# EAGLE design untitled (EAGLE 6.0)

## Sheet 1 of 3: NAP a SERVO
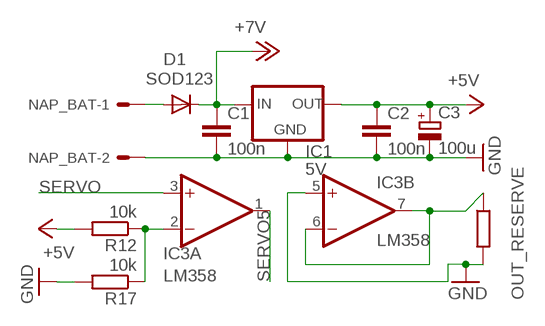
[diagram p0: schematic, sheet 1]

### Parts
C1  100n  C-EUC0805K  [C0805K]
C2  100n  C-EUC0805K  [C0805K]
C3  100u  CPOL-EUE2-5  [E2-5]
D1  SOD123  CGRM4001-G  [SOD-123_MINI-SMA]
IC1  5V  78XXL  [78XXL]
IC3  LM358  TL072D  [SO08]
NAP_BAT  22-27-2021-02  [6410-02]
OUT_RESERVE  R-EU_R0805  [R0805]
R12  10k  R-EU_R0805  [R0805]
R17  10k  R-EU_R0805  [R0805]

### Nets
+7V: C1.1 D1.C IC1.IN ; also sheet 2
GND: C1.2 C2.2 C3.- IC1.GND IC3.5(B:+IN) NAP_BAT.2 OUT_RESERVE.2 R17.2 ; also sheet 2,3
N$2: D1.A NAP_BAT.1
N$6: IC3.6(B:-IN) IC3.7(B:OUT) OUT_RESERVE.1
N$14: IC3.2(A:-IN) R12.1 R17.1
SERVO: IC3.3(A:+IN) ; also sheet 2
SERVO5: IC3.1(A:OUT) ; also sheet 2
VCC: C2.1 C3.+ IC1.OUT R12.2 ; supply symbol labelled +5V ; also sheet 2,3

## Sheet 2 of 3: HEADER_IO
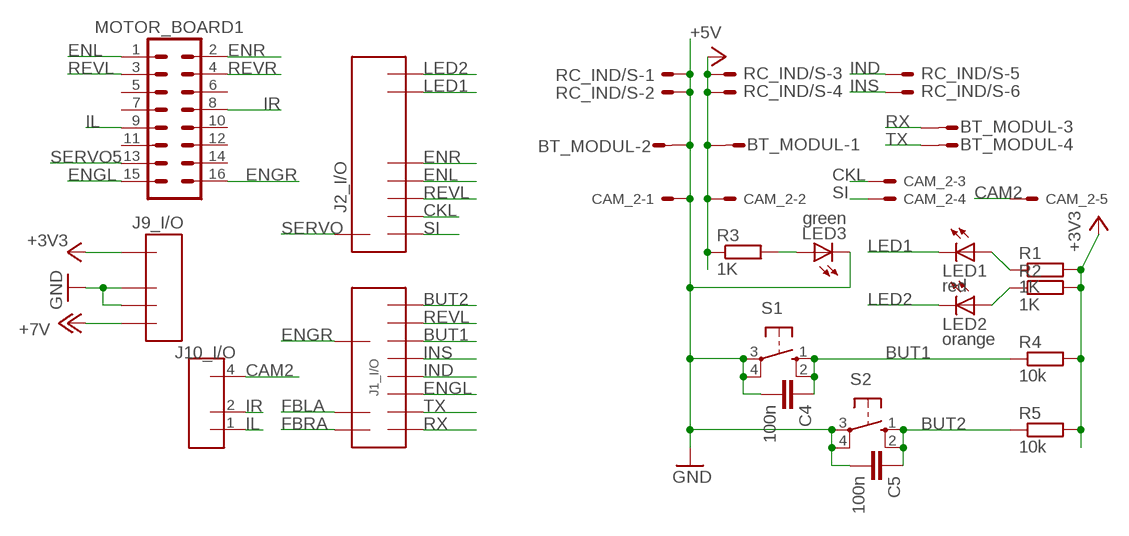
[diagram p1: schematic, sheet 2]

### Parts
BT_MODUL  M04S  [04P]
C4  100n  C-EUC0805K  [C0805K]
C5  100n  C-EUC0805K  [C0805K]
CAM_2  22-27-2051-05  [6410-05]
J1_I/O  DOLNE  [DOLNE]
J2_I/O  HORNE  [HORNE]
J9_I/O  NAP  [NAP]
J10_I/O  ANALOG  [ANALOG]
LED1  red  LED3MM  [LED3MM]
LED2  orange  LED3MM  [LED3MM]
LED3  green  LED3MM  [LED3MM]
MOTOR_BOARD1  ML16  [ML16]
R1  1K  R-EU_R0805  [R0805]
R2  1K  R-EU_R0805  [R0805]
R3  1K  R-EU_R0805  [R0805]
R4  10k  R-EU_R0805  [R0805]
R5  10k  R-EU_R0805  [R0805]
RC_IND/S  ML6E  [ML6]
S1  10-XX  [B3F-10XX]
S2  10-XX  [B3F-10XX]

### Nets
+3V3: J9_I/O.1 R1.2 R2.2 R4.2 R5.2
+7V: J9_I/O.4 ; also sheet 1
BUT1: C4.1 J1_I/O.P$9 R4.1 S1.1(S) S1.2(S1)
BUT2: C5.1 J1_I/O.P$11 R5.1 S2.1(S) S2.2(S1)
CAM2: CAM_2.5 J10_I/O.4
CKL: CAM_2.3 J2_I/O.P$3
ENGL: J1_I/O.P$5 MOTOR_BOARD1.15
ENGR: J1_I/O.P$8 MOTOR_BOARD1.16
ENL: J2_I/O.P$5 MOTOR_BOARD1.1
ENR: J2_I/O.P$6 MOTOR_BOARD1.2
FBLA: J1_I/O.P$3 ; also sheet 3
FBRA: J1_I/O.P$1 ; also sheet 3
GND: BT_MODUL.2 C4.2 C5.2 CAM_2.1 J9_I/O.2 J9_I/O.3 LED3.K(C) RC_IND/S.1 RC_IND/S.2 S1.3(P) S1.4(P1) S2.3(P) S2.4(P1) ; also sheet 1,3
IL: J10_I/O.1 MOTOR_BOARD1.9
IND: J1_I/O.P$6 RC_IND/S.5
INS: J1_I/O.P$7 RC_IND/S.6
IR: J10_I/O.2 MOTOR_BOARD1.8
LED1: J2_I/O.P$7 LED1.K(C)
LED2: J2_I/O.P$8 LED2.K(C)
N$1: LED1.A R1.1
N$15: LED2.A R2.1
N$16: LED3.A R3.2
REVL: J1_I/O.P$10 J2_I/O.P$4 MOTOR_BOARD1.3
REVR: MOTOR_BOARD1.4
RX: BT_MODUL.3 J1_I/O.P$2
SERVO: J2_I/O.P$1 ; also sheet 1
SERVO5: MOTOR_BOARD1.13 ; also sheet 1
SI: CAM_2.4 J2_I/O.P$2
TX: BT_MODUL.4 J1_I/O.P$4
VCC: BT_MODUL.1 CAM_2.2 R3.1 RC_IND/S.3 RC_IND/S.4 ; supply symbol labelled +5V ; also sheet 1,3
Unconnected: MOTOR_BOARD1.5 MOTOR_BOARD1.6 MOTOR_BOARD1.7 MOTOR_BOARD1.10 MOTOR_BOARD1.11 MOTOR_BOARD1.12 MOTOR_BOARD1.14

## Sheet 3 of 3: CNY70
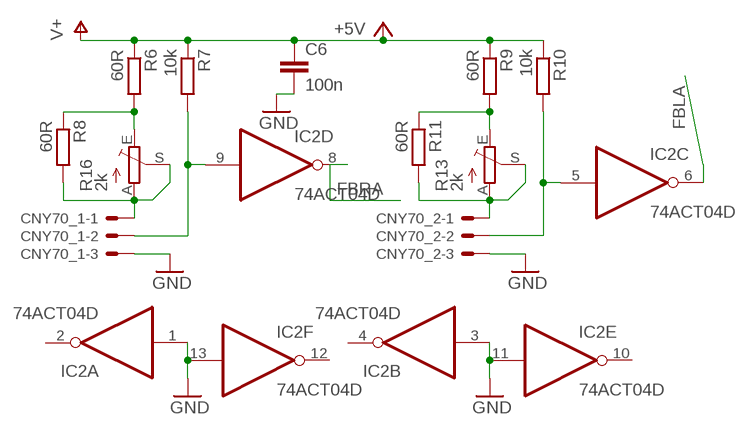
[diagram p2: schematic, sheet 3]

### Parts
C6  100n  C-EUC0805K  [C0805K]
CNY70_1  22-27-2031-03  [6410-03]
CNY70_2  22-27-2031-03  [6410-03]
IC2  74ACT04D  [SO14]
R6  60R  R-EU_R0603  [R0603]
R7  10k  R-EU_R0603  [R0603]
R8  60R  R-EU_R0603  [R0603]
R9  60R  R-EU_R0603  [R0603]
R10  10k  R-EU_R0603  [R0603]
R11  60R  R-EU_R0603  [R0603]
R13  2k  TRIM_EU-CA6V  [CA6V]
R16  2k  TRIM_EU-CA6V  [CA6V]

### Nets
FBLA: IC2.6(C:O) ; also sheet 2
FBRA: IC2.8(D:O) ; also sheet 2
GND: C6.2 CNY70_1.3 CNY70_2.3 IC2.1(A:I) IC2.3(B:I) IC2.11(E:I) IC2.13(F:I) ; also sheet 1,2
N$3: R9.2 R11.1 R13.E
N$4: R6.2 R8.1 R16.E
N$5: CNY70_2.1 R11.2 R13.A R13.S
N$8: CNY70_1.1 R8.2 R16.A R16.S
N$9: CNY70_1.2 IC2.9(D:I) R7.2
N$10: CNY70_2.2 IC2.5(C:I) R10.2
VCC: C6.1 R6.1 R7.1 R9.1 R10.1 ; supply symbol labelled V+, +5V ; also sheet 1,2
Unconnected: IC2.2(A:O) IC2.4(B:O) IC2.10(E:O) IC2.12(F:O)

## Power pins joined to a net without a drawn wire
GND: IC2.7(P:GND) IC3.4(P:V-)
VCC: IC2.14(P:VCC) IC3.8(P:V+)

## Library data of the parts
BT_MODUL = con-amp-quick:M04S: AMP QUICK CONNECTOR; OC_FARNELL: unknown; OC_NEWARK: unknown
C1 C2 C4-C6 = rcl:C-EU: CAPACITOR, European symbol
C3 = rcl:CPOL-EU: POLARIZED CAPACITOR, European symbol
CAM_2 = con-molex:22-?-05: CONNECTOR wire to board 2.54 mm (.1 inch) pitch header; OC_FARNELL: unknown; OC_NEWARK: unknown
CNY70_1 CNY70_2 = con-molex:22-?-03: CONNECTOR wire to board 2.54 mm (.1 inch) pitch header; OC_FARNELL: unknown; OC_NEWARK: unknown
D1 = diode:CGRM400*-G: Molded plasitc,JEDEC SOD-123/Mini SMA
IC1 = v-reg:78XXL: VOLTAGE REGULATOR
IC2 = 74xx-eu:74*04: Hex INVERTER
IC3 = linear:TL072: OP AMP
J1_I/O = con-tfc:DOLNE
J2_I/O = con-tfc:HORNE
J9_I/O = con-tfc:NAP
J10_I/O = con-tfc:ANALOG
LED1-LED3 = led:LED: LED
MOTOR_BOARD1 = con-ml:ML16: HARTING; OC_FARNELL: unknown; OC_NEWARK: unknown
NAP_BAT = con-molex:22-?-02: CONNECTOR; OC_FARNELL: unknown; OC_NEWARK: unknown
OUT_RESERVE R1-R12 R17 = rcl:R-EU_: RESISTOR, European symbol
R13 R16 = pot:TRIM_EU-: POTENTIOMETER
RC_IND/S = con-ml:ML6E: HARTING; OC_FARNELL: unknown; OC_NEWARK: unknown
S1 S2 = switch-omron:10-XX: OMRON SWITCH; MPN: B3F-1000; OC_FARNELL: 176432; OC_NEWARK: 36M3542

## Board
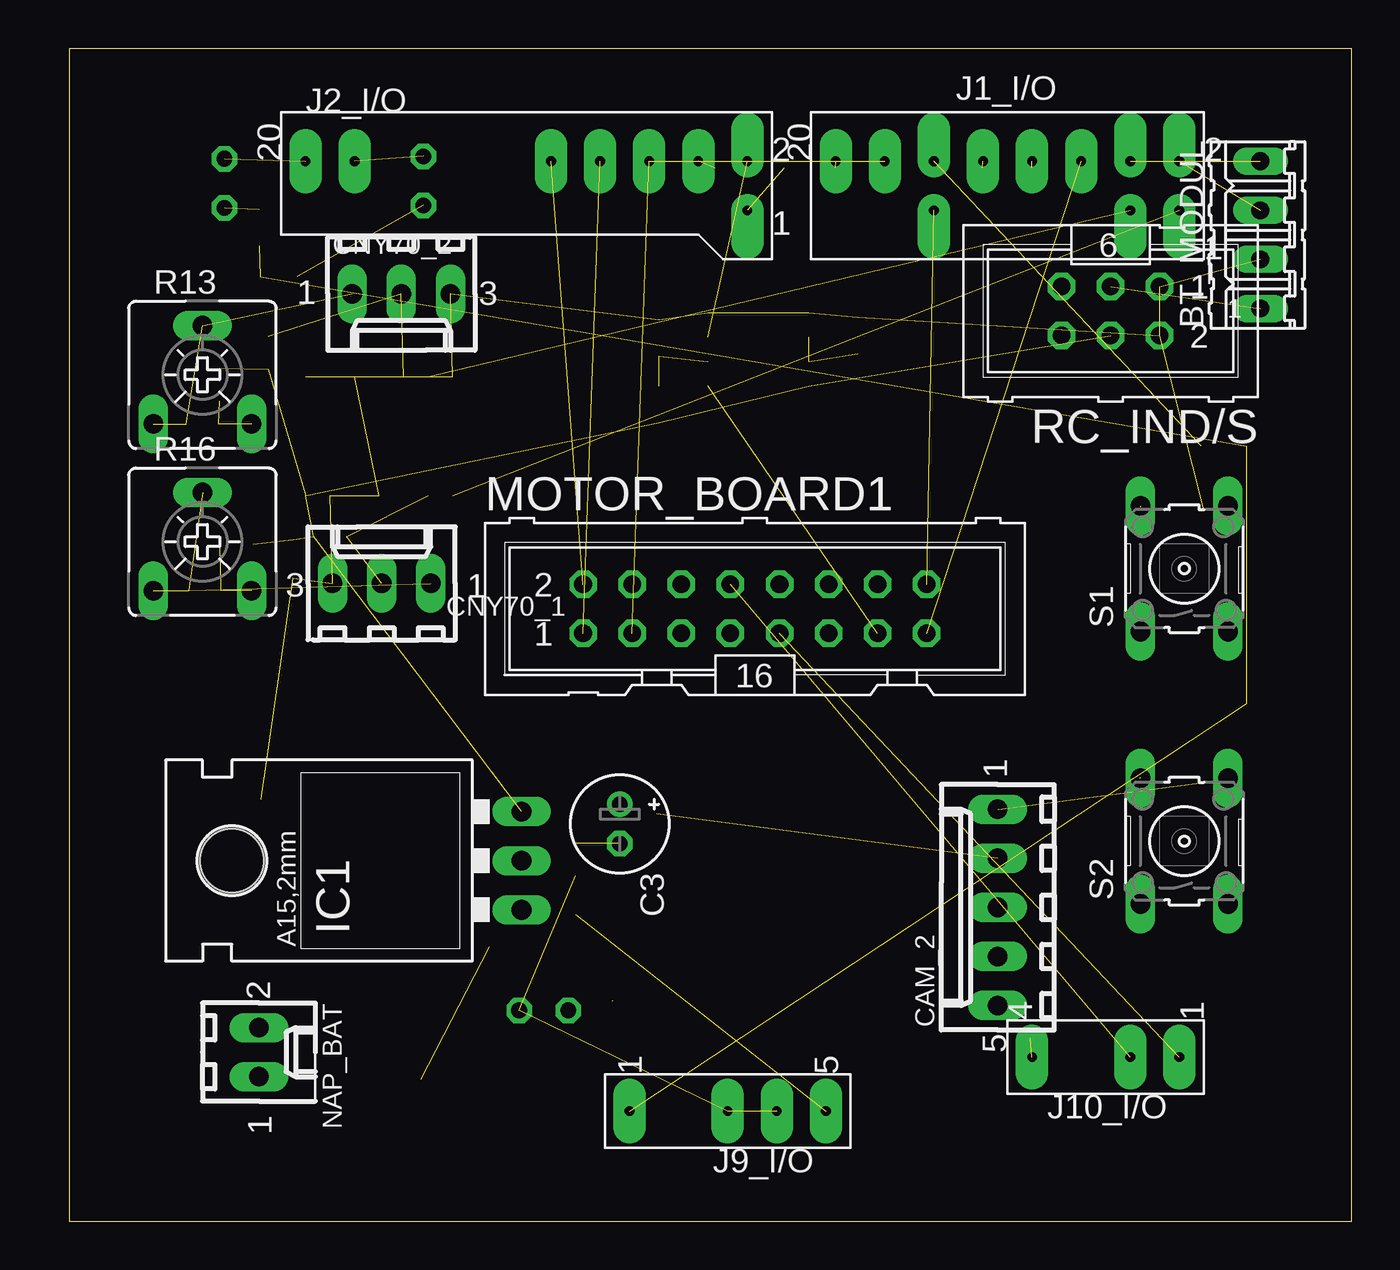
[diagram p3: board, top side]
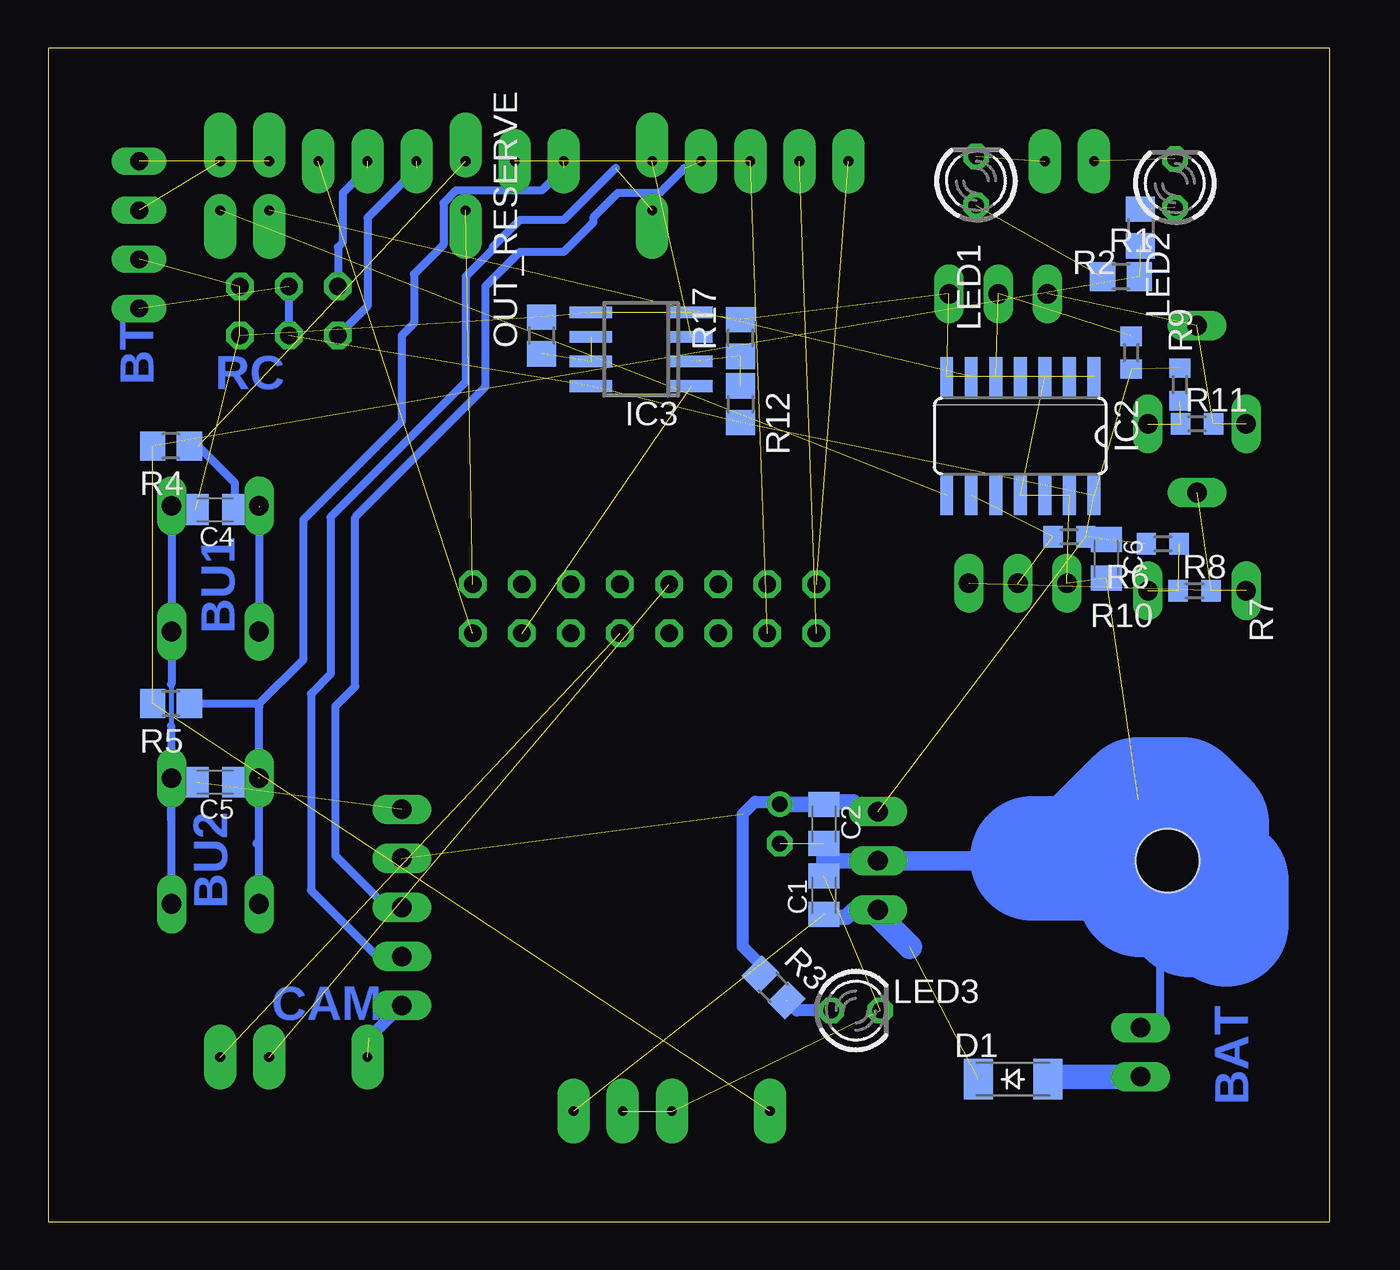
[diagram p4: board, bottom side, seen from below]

Size 66.29 x 60.71 mm. Coordinates in mm from the lower left corner, seen from the top.
Outline: 0,60.71 66.29,60.71 66.29,0 0,0 0,60.71
Copper layers (1*16): Top 0.035mm / dielectric 1.5mm / Bottom 0.035mm
Design rules: minimum track width 10mil, minimum drill 24mil, track to track 8mil, track to pad 8mil, pad to pad 8mil, via to via 8mil, smd to smd 8mil, copper to edge 40mil, drill to drill 8mil, minimum pad ring 10mil, minimum via ring 8mil, stop-mask expansion 4mil, vias tented up to drill 0mil, thermal gap 10mil

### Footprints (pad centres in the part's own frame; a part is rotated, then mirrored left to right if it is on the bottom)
04P = drill 0.914 long: 1 -3.81,0; 2 -1.27,0; 3 1.27,0; 4 3.81,0
C0805K = smd 1.3 x 1.6: 1 -1,0; 2 1,0
E2-5 = drill 0.813 pad 1.27: + -1.016,0 | drill 0.813 pad 1.27 octagon: - 1.016,0
6410-05 = drill 1.016 long: 1 5.08,0; 2 2.54,0; 3 0,0; 4 -2.54,0; 5 -5.08,0
6410-03 = drill 1.016 long: 1 2.54,0; 2 0,0; 3 -2.54,0
SOD-123_MINI-SMA = smd 1.5 x 2.1: A 1.8,0; C -1.8,0
78XXL = drill 1.016 long: GND 0,-3.81; IN -2.54,-3.81; OUT 2.54,-3.81 | hole 3.302: 0,11.176
SO14 = smd 0.66 x 2.032: 1 -3.81,-3.073; 2 -2.54,-3.073; 3 -1.27,-3.073; 4 0,-3.073; 5 1.27,-3.073; 6 2.54,-3.073; 7 3.81,-3.073; 8 3.81,3.073; 9 2.54,3.073; 10 1.27,3.073; 11 0,3.073; 12 -1.27,3.073; 13 -2.54,3.073; 14 -3.81,3.073
SO08 = smd 0.6 x 2.2: 1 -1.905,-2.6; 2 -0.635,-2.6; 3 0.635,-2.6; 4 1.905,-2.6; 5 1.905,2.6; 6 0.635,2.6; 7 -0.635,2.6; 8 -1.905,2.6
DOLNE = drill 0.5 pad 1.676 offset: P$1 8.89,-1.27; P$2 8.89,1.27; P$3 6.35,-1.27; P$4 6.35,1.27; P$8 -3.81,-1.27; P$9 -3.81,1.27 | drill 0.5 pad 1.676 long: P$5 3.81,1.27; P$6 1.27,1.27; P$7 -1.27,1.27; P$10 -6.35,1.27; P$11 -8.89,1.27
HORNE = drill 0.5 pad 1.676 offset: P$1 8.89,1.27; P$2 8.89,-1.27 | drill 0.5 pad 1.676 long: P$3 6.35,1.27; P$4 3.81,1.27; P$5 1.27,1.27; P$6 -1.27,1.27; P$7 -11.43,1.27; P$8 -13.97,1.27
NAP = drill 0.5 pad 1.676 long: 1 0,5.08; 2 0,0; 3 0,-2.54; 4 0,-5.08
ANALOG = drill 0.5 pad 1.676 long: 1 0,-3.81; 2 0,-1.27; 4 0,3.81
LED3MM = drill 0.813 octagon: A -1.27,0; K 1.27,0
ML16 = drill 0.914 octagon: 1 -8.89,-1.27; 2 -8.89,1.27; 3 -6.35,-1.27; 4 -6.35,1.27; 5 -3.81,-1.27; 6 -3.81,1.27; 7 -1.27,-1.27; 8 -1.27,1.27; 9 1.27,-1.27; 10 1.27,1.27; 11 3.81,-1.27; 12 3.81,1.27; 13 6.35,-1.27; 14 6.35,1.27; 15 8.89,-1.27; 16 8.89,1.27
6410-02 = drill 1.016 long: 1 1.27,0; 2 -1.27,0
R0805 = smd 1.3 x 1.5: 1 -0.95,0; 2 0.95,0
R0603 = smd 1 x 1.1: 1 -0.85,0; 2 0.85,0
CA6V = drill 1.016 long: A -2.54,-2.54; E 2.54,-2.54; S 0,2.54
ML6 = drill 0.914 octagon: 1 -2.54,-1.27; 2 -2.54,1.27; 3 0,-1.27; 4 0,1.27; 5 2.54,-1.27; 6 2.54,1.27
B3F-10XX = drill 1.016 long: 1 -3.251,2.261; 2 3.251,2.261; 3 -3.251,-2.261; 4 3.251,-2.261

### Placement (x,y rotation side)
BT_MODUL  61.6,51.05 90 top
C1  26.16,16.89 90 bottom
C2  26.16,20.57 270 bottom
C3  28.45,20.57 270 top
C4  57.66,36.83 180 bottom
C5  57.66,22.73 180 bottom
C6  11.56,34.29 270 bottom
CAM_2  48.01,16.26 90 top
CNY70_1  16.13,33.02 0 top
CNY70_2  17.14,48.01 180 top
D1  16.38,7.37 0 bottom
IC1  19.56,18.67 90 top
IC2  16,40.64 180 bottom
IC3  35.62,45.13 90 bottom
J1_I/O  48.51,53.59 0 top
J2_I/O  26.16,53.59 0 top
J9_I/O  34.04,5.71 90 top
J10_I/O  53.59,8.51 90 top
LED1  18.29,53.85 90 bottom
LED2  8,53.72 90 bottom
LED3  24.51,10.92 0 bottom
MOTOR_BOARD1  35.44,31.7 0 top
NAP_BAT  9.78,8.76 270 top
OUT_RESERVE  40.77,45.85 90 bottom
R1  10.79,48.89 0 bottom
R2  9.78,51.43 270 bottom
R3  28.78,12.12 315 bottom
R4  59.94,40.13 180 bottom
R5  59.94,26.8 180 bottom
R6  8.63,35.07 0 bottom
R7  13.46,35.43 180 bottom
R8  6.98,32.64 0 bottom
R9  7.75,43.31 270 bottom
R10  10.27,44.96 90 bottom
R11  6.86,41.27 0 bottom
R12  30.48,42.29 270 bottom
R13  6.86,43.81 0 top
R16  6.86,35.18 0 top
R17  30.48,45.72 90 bottom
RC_IND/S  53.85,47.12 180 top
S1  57.66,33.78 90 top
S2  57.66,19.69 90 top

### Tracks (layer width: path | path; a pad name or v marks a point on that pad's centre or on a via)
+3V3  (4 unrouted)
+7V  (2 unrouted)
  Bottom 0.813: IC1.IN 24.64,16.13 25.02,15.75 26.02,15.75 C1.1
  Bottom 1.27: IC1.IN 23.37,15.88 21.72,14.22
BUT1  (2 unrouted)
  Bottom 0.406: 55.37,36.96 55.5,36.83 C4.1 56.64,36.85 56.64,38.23 58.55,40.13 R4.1 | S1.2 S1.1
BUT2  (3 unrouted)
  Bottom 0.406: 39.6,54.5 40.77,53.34 45.21,53.34 45.85,52.7 45.85,50.55 47.37,49.02 47.37,46.48 48.01,45.85 48.01,41.4 53.09,36.32 53.09,29.08 55.37,26.8 55.37,26.67 | S2.1 55.4,19.69 | 55.4,19.69 S2.2 56.57,22.94 56.64,22.86 56.64,22.73 56.77,22.73 | 55.52,19.56 55.4,19.69 | 55.37,22.99 55.37,26.67 | R5.1 55.5,26.8 55.37,26.67
CAM2  (1 unrouted)
  Bottom 0.61: 49.69,9.5 CAM_2.5
CKL  (1 unrouted)
  Bottom 0.406: 33.38,54.5 34.67,53.21 36.83,53.21 38.1,51.94 38.1,51.69 39.62,50.16 41.91,50.16 43.69,48.39 43.69,43.18 50.42,36.45 50.42,27.69 51.44,26.67 51.44,18.92 48.77,16.26 CAM_2.3
ENGL  (1 unrouted)
ENGR  (1 unrouted)
ENL  (1 unrouted)
ENR  (1 unrouted)
FBLA  (1 unrouted)
FBRA  (1 unrouted)
GND  (21 unrouted)
  Bottom 0.254: 59.94,27.81 59.94,25.65
  Bottom 0.406: 59.94,20.83 59.94,22.73 | 59.94,22.73 59.94,22.91 S2.4 | C5.2 59.72,22.73 S2.4 | C4.2 59.72,36.83 S1.4 S1.3 59.92,27.84 59.94,27.81 | NAP_BAT.2 8.76,10.03 8.76,16.89 8,16.89 8,19.69 6.6,19.69 | S2.3 59.92,22.71 59.94,22.73 | 59.94,25.65 59.94,23.24 59.82,23.11 59.82,23.04 S2.4
  Bottom 0.61: 28.7,19.3 C3.-
  Bottom 0.813: IC1.GND 26.16,18.67 | 26.16,18.67 C2.2 26.18,19.56 | 26.16,18.67 C1.2
  Bottom 1.016: IC1.GND 15.49,18.67 15.37,18.8
  Bottom 6.452: 15.37,18.8 12.95,18.8 9.91,21.84 7.62,21.84 6.35,20.57 6.35,20.32 9.78,16.89 8.76,16.89 8.26,16.89 7.24,15.88 7.11,15.88 5.33,17.65 5.33,15.37
IL  (1 unrouted)
IND  (1 unrouted)
  Bottom 0.406: 49.76,54.5 51.05,53.21 51.05,50.67 51.31,50.42 RC_IND/S.5
INS  (1 unrouted)
  Bottom 0.406: 47.22,54.5 49.78,51.94 49.78,47.37 RC_IND/S.6
IR  (1 unrouted)
LED1  (1 unrouted)
LED2  (1 unrouted)
N$1  (1 unrouted)
N$2
  Bottom 1.27: NAP_BAT.1 14.46,7.49 D1.A
N$3  (2 unrouted)
N$4  (2 unrouted)
N$5  (3 unrouted)
N$6  (2 unrouted)
N$8  (3 unrouted)
N$9  (2 unrouted)
N$10  (2 unrouted)
N$14  (2 unrouted)
N$15  (1 unrouted)
N$16  (1 unrouted)
  Bottom 0.61: LED3.A 27.56,10.92 28.07,11.43
REVL  (2 unrouted)
RX  (1 unrouted)
SERVO  (1 unrouted)
SERVO5  (1 unrouted)
SI  (1 unrouted)
  Bottom 0.406: 36.94,54.5 39.62,51.82 41.91,51.82 43.31,50.42 43.31,50.29 44.7,48.89 44.7,43.43 51.69,36.45 51.69,28.32 52.71,27.3 52.71,17.14 49.28,13.72 CAM_2.4
TX  (1 unrouted)
VCC  (11 unrouted)
  Bottom 0.406: RC_IND/S.3 RC_IND/S.4
  Bottom 0.61: C3.+ 28.57,21.72 29.72,21.72 30.35,21.08 30.35,14.22 29.45,13.32 R3.1
  Bottom 0.813: IC1.OUT 24.13,21.21 24.64,21.72 26.02,21.72 C2.1 28.43,21.57 C3.+

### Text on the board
Bottom: BT | RC | BU1 | BU2 | BAT | CAM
